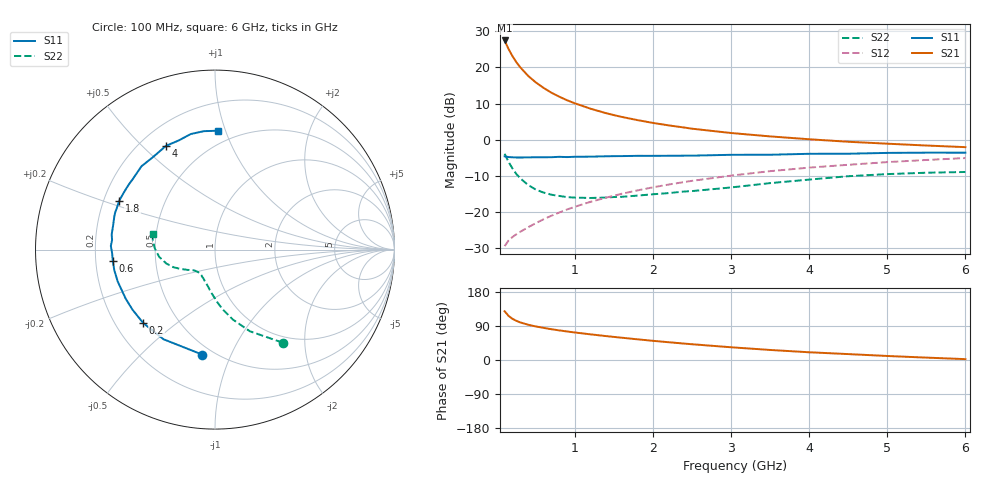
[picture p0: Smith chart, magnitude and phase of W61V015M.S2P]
! SIEMENS Small Signal Semiconductors
! BFR193W
! Si NPN RF Bipolar Junction Transistor in SOT323
! VCE = 1 V  IC = 15 mA
! Common Emitter S-Parameters:  September  1992
# GHz  S  MA  R  50
!  f  S11  S21  S12  S22
! GHz  MAG  ANG  MAG  ANG  MAG  ANG  MAG  ANG
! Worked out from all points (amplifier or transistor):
!   28 points, 100 MHz to 6 GHz, reference 50 ohm
!   highest |S21| = 27.4 dB at 100 MHz (marker M1)
!   |S21| within 3 dB of that: start of sweep to 166.5 MHz
!   unconditionally stable (mu >= 1): 793 MHz to 2.734 GHz
!   at 300 MHz: K = 0.70, MSG = 22.7 dB, |S12| = -25.4 dB
!   at 1.5 GHz: K = 1.05, MAG = 9.8 dB, |S12| = -15.5 dB
!   at 6 GHz: K = 0.94, MSG = 1.5 dB, |S12| = -5.1 dB
!   S11 on the Smith chart (normalised r, x): 100 MHz: 0.44, -0.79; 200 MHz: 0.32, -0.38; 600 MHz: 0.27, -0.05; 1.8 GHz: 0.26, +0.22; 4 GHz: 0.30, +0.59; 6 GHz: 0.40, +0.94
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0.1  0.5897 -96.8  23.57 128.6  0.0338 54.2  0.6407 -54.0
0.15  0.576 -119.9  17.99 116.6  0.0404 49.7  0.4945 -66.9
0.2  0.5721 -134.4  14.33 108.7  0.0452 48.9  0.4018 -75.7
0.25  0.5686 -144.2  11.82 103.4  0.0493 49.5  0.3365 -82.6
0.3  0.5677 -151.3  10.04 99.2  0.0534 50.7  0.294 -87.4
0.4  0.5704 -161.8  7.658 93.1  0.0616 53.7  0.2371 -95.6
0.5  0.5727 -168.4  6.195 88.5  0.0703 56.4  0.2045 -101.8
0.6  0.5728 -173.8  5.2 84.7  0.0797 58.5  0.186 -107.5
0.7  0.5737 -178.1  4.462 81.2  0.0891 60.1  0.1738 -111.5
0.8  0.5807 178.0  3.937 78.1  0.0987 61.4  0.1671 -115.3
0.9  0.5759 174.7  3.511 75.3  0.1087 62.2  0.1611 -118.4
1  0.5818 171.7  3.188 72.6  0.1186 62.7  0.1586 -121.1
1.2  0.5838 166.2  2.685 67.7  0.1386 63.1  0.1567 -126.9
1.5  0.5934 159.7  2.19 60.9  0.1684 63.0  0.1615 -132.6
1.8  0.5991 153.1  1.869 54.6  0.1994 61.9  0.169 -137.3
2.2  0.6004 145.1  1.58 46.9  0.2402 60.0  0.183 -141.7
3  0.6192 131.4  1.239 33.6  0.3192 54.2  0.2191 -150.5
3.5  0.6205 123.8  1.112 26.5  0.368 50.0  0.2515 -157.0
4  0.6393 115.3  1.016 20.4  0.4118 45.5  0.2815 -163.9
4.5  0.6409 108.3  0.938 15.6  0.4506 41.2  0.3133 -172.5
5.5  0.6628 95.4  0.832 6.3  0.5254 32.3  0.35 171.6
6  0.6625 88.5  0.79 2.3  0.5586 27.6  0.3584 166.3
